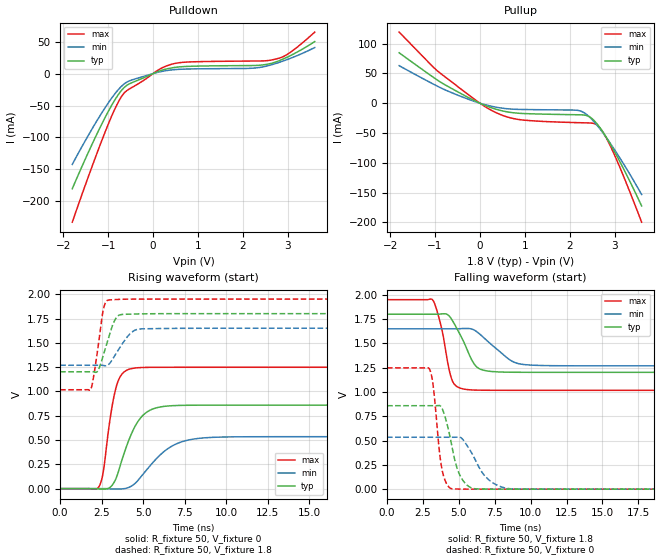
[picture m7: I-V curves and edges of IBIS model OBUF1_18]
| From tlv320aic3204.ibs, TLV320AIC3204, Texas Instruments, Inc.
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[Model]   OBUF1_18
Model_type  Output
Vref =   0
|Rref =   50
Cref =   10p
Vmeas =   0.9
| variable   typ   min   max
C_comp   3.00pF   1.69pF   4.50pF
| C_pullup   3.39pF   1.78pF   4.50pF
| C_pulldown   2.61pF   1.69pF   3.33pF
[Temperature Range]   40   100   -40
| Ambient temperature   25   85   -40
[Voltage range]   1.8   1.65   1.95
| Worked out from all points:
|   slope of the pulldown table from 0 to 0.27 V, typ, clamps not added: 40.3 ohm
|   slope of the pullup table from 0 to 0.27 V, typ, clamps not added: 33.7 ohm
|   rising waveform, R_fixture 50, V_fixture 0: 20-80 % time 1.17ns typ, 1.84ns min, 645ps max; typ from 0 V to 0.859 V
|   falling waveform, R_fixture 50, V_fixture 1.8: 20-80 % time 1.17ns typ, 1.79ns min, 751ps max; typ from 1.8 V to 1.2 V
|   rising waveform, R_fixture 50, V_fixture 1.8: 20-80 % time 647ps typ, 896ps min, 459ps max; typ from 1.2 V to 1.8 V
|   falling waveform, R_fixture 50, V_fixture 0: 20-80 % time 837ps typ, 1.34ns min, 506ps max; typ from 0.859 V to 0 V
[Pulldown]
| OBUF1_18
|   Voltage   I(typ)   I(min)   I(max)
-1.8V     -180.3mA   -142.2mA   -232.7mA
-1.35V    -109.3mA   -85.56mA   -143.7mA
-985mV    -57.59mA   -44.63mA   -76.91mA
-755mV    -31.02mA   -23.63mA   -41.97mA
-590mV    -18.7mA    -13.63mA   -26.95mA
145mV     4.06mA     2.627mA    6.836mA
480mV     9.604mA    6.154mA    15.76mA
2.215V    12.57mA    8.391mA    19.63mA
2.55V     14.72mA    12.11mA    20.3mA
2.815V    20.34mA    17.71mA    24.34mA
3.105V    29.81mA    25.18mA    35.75mA
3.6V      50.11mA    40.73mA    64.94mA
[Pullup]
| OBUF1_18
|   Voltage   I(typ)   I(min)   I(max)
-1.8V     84.57mA    62.96mA    119.3mA
-935mV    38.13mA    28.07mA    53.42mA
-140mV    5.029mA    3.465mA    7.627mA
355mV     -10.02mA   -6.6mA     -15.69mA
910mV     -17.05mA   -10.44mA   -27.79mA
2.19V     -19.37mA   -12.18mA   -32.61mA
2.42V     -21.98mA   -21.78mA   -33.06mA
2.61V     -34.94mA   -37.22mA   -36.85mA
2.76V     -50.81mA   -51.93mA   -51.23mA
2.96V     -76.18mA   -73.74mA   -80.73mA
3.23V     -114.8mA   -105.7mA   -128.5mA
3.6V      -172.3mA   -153.2mA   -199.5mA
[Ramp]
| OBUF1_18
| variable   typ   min   max
dV/dt_r   0.52/1.17E-09   0.32/1.85E-09   0.75/6.49E-10
dV/dt_f   0.36/1.18E-09   0.23/1.81E-09   0.56/7.60E-10
R_load = 50
[Rising Waveform]
| OBUF1_18
R_fixture =   50
C_fixture =   0
L_fixture =   0
V_fixture =   0
V_fixture_min = 0
V_fixture_max = 0
|   Time   V(typ)   V(min)   V(max)
0s        1.707nV    16.08nV    574pV
2.33ns    -3.527mV   -25.58uV   18.12mV
2.58ns    -4.954mV   311.9uV    156.5mV
3.055ns   20.4mV     -3.009mV   771.1mV
3.42ns    129.7mV    -3.852mV   1.071V
4.565ns   657.6mV    62.45mV    1.242V
5.38ns    804mV      228mV      1.247V
6.69ns    852.4mV    433.5mV    1.248V
9.225ns   858.6mV    527.7mV    1.248V
70ns      858.8mV    534.2mV    1.248V
[Falling Waveform]
| OBUF1_18
R_fixture =   50
C_fixture =   0
L_fixture =   0
V_fixture =   1.8
V_fixture_min = 1.65
V_fixture_max = 1.95
|   Time   V(typ)   V(min)   V(max)
0s        1.8V       1.65V      1.95V
3.175ns   1.8V       1.65V      1.948V
3.755ns   1.802V     1.65V      1.683V
4.53ns    1.74V      1.65V      1.121V
5.665ns   1.404V     1.653V     1.024V
6.135ns   1.276V     1.631V     1.02V
6.64ns    1.227V     1.571V     1.018V
8.705ns   1.203V     1.317V     1.017V
10.32ns   1.202V     1.274V     1.017V
70ns      1.202V     1.269V     1.017V
[Rising Waveform]
| OBUF1_18
R_fixture =   50
C_fixture =   0
L_fixture =   0
V_fixture =   1.8
V_fixture_min = 1.65
V_fixture_max = 1.95
|   Time   V(typ)   V(min)   V(max)
0s        1.202V     1.269V     1.017V
1.835ns   1.202V     1.269V     1.018V
2.25ns    1.207V     1.269V     1.417V
2.605ns   1.376V     1.267V     1.845V
2.775ns   1.471V     1.263V     1.927V
3.015ns   1.606V     1.295V     1.942V
3.53ns    1.782V     1.434V     1.947V
4.29ns    1.795V     1.605V     1.949V
4.99ns    1.798V     1.644V     1.95V
70ns      1.8V       1.65V      1.95V
[Falling Waveform]
| OBUF1_18
R_fixture =   50
C_fixture =   0
L_fixture =   0
V_fixture =   0
V_fixture_min = 0
V_fixture_max = 0
|   Time   V(typ)   V(min)   V(max)
0s        858.8mV    534.2mV    1.248V
2.955ns   858.8mV    534.2mV    1.237V
3.22ns    858.7mV    534.2mV    1.056V
3.82ns    835.1mV    534.2mV    208.8mV
4.54ns    424mV      534mV      3.61mV
5.005ns   165.3mV    536.9mV    1.329mV
5.685ns   28.36mV    422.9mV    321.8uV
6.985ns   922.2uV    109.7mV    29.32uV
8.695ns   83.87uV    3.028mV    2.35uV
70ns      1.625nV    16.23nV    533.1pV
